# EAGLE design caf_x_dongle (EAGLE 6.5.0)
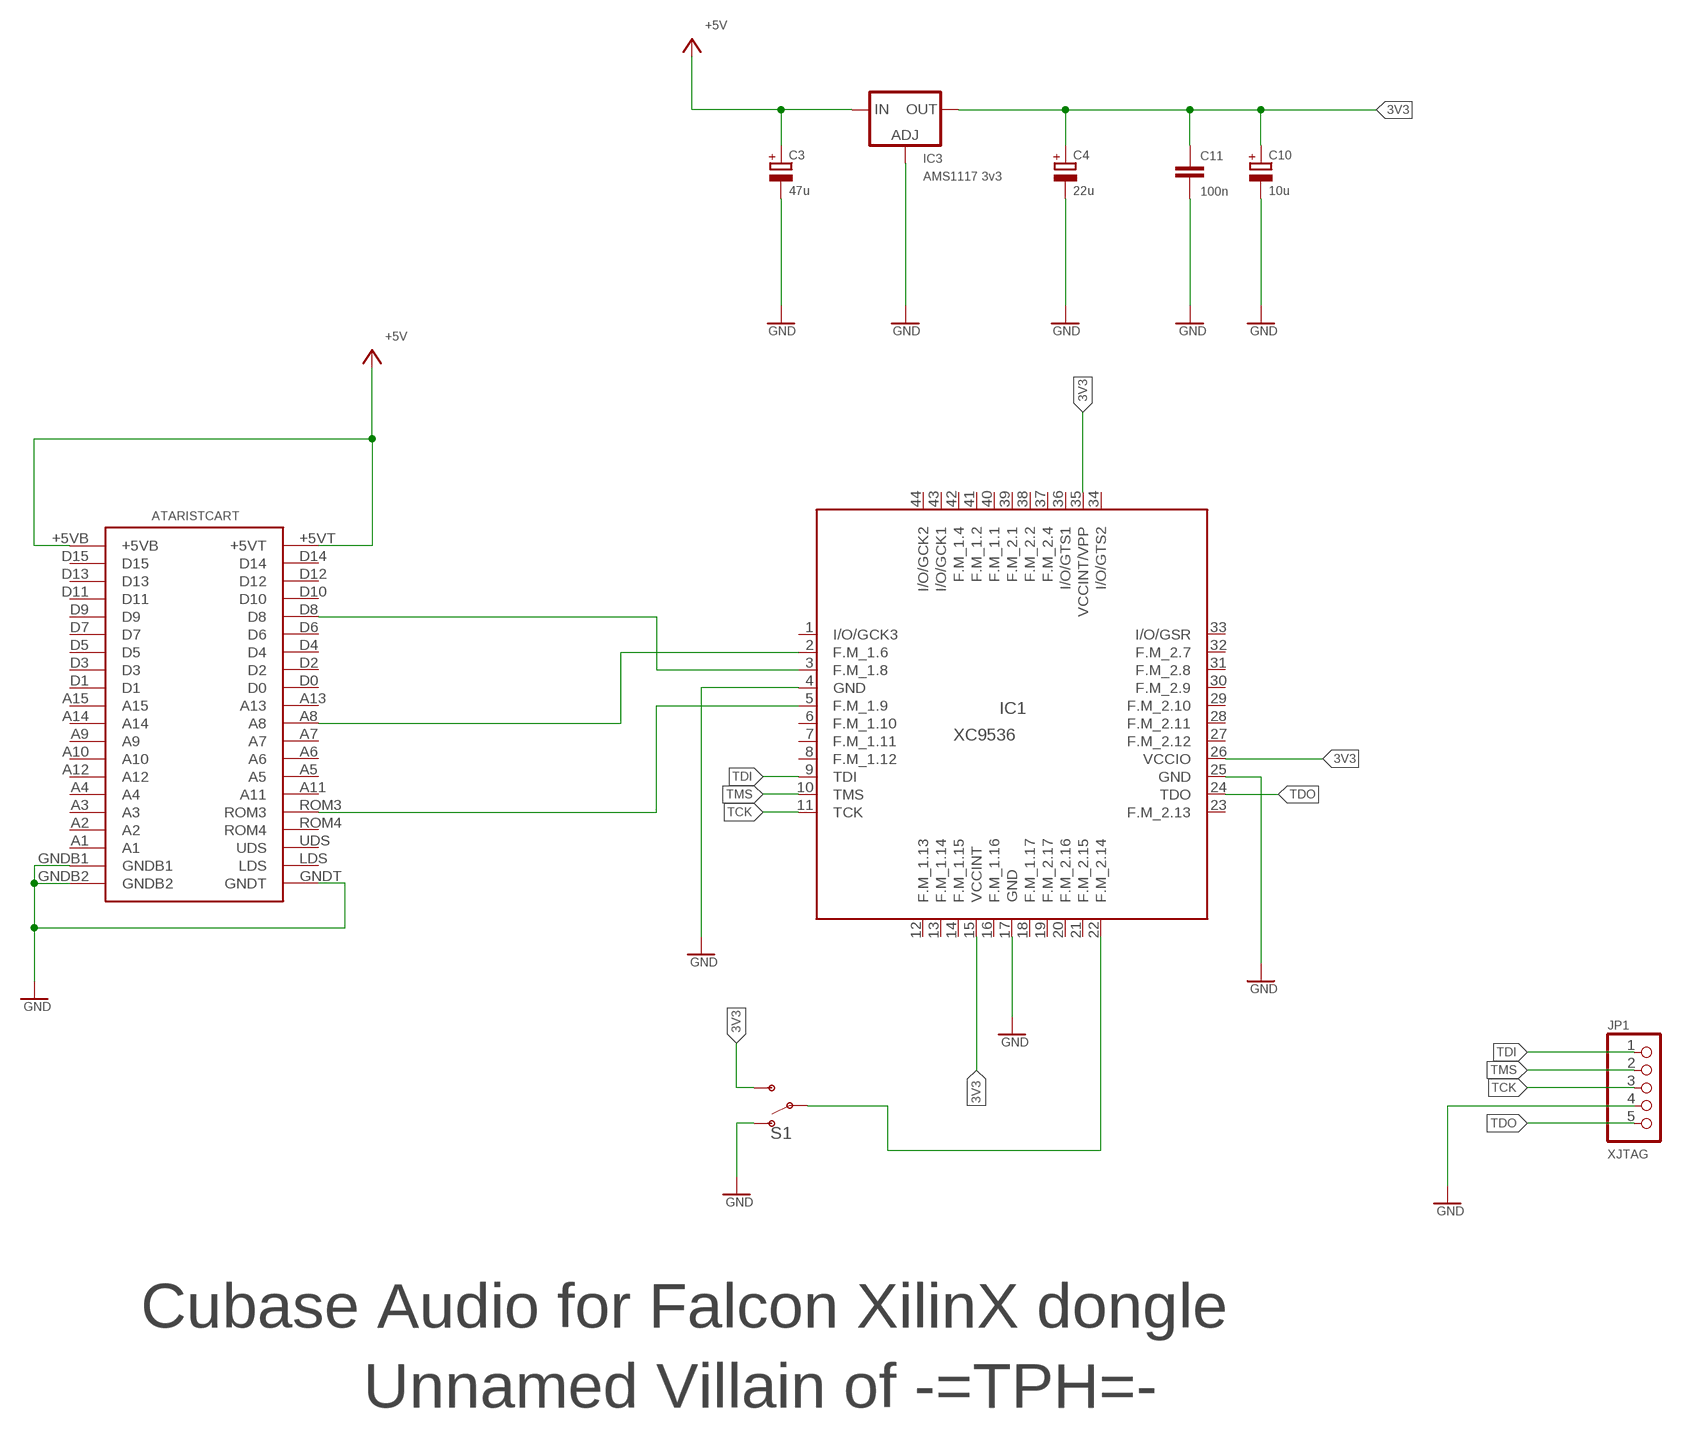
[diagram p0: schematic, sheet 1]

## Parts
C3  47u  CPOL-EUSMCD  [SMC_D]
C4  22u  CPOL-EUSMCD  [SMC_D]
C10  10u  CPOL-EUSMCB  [SMC_B]
C11  100n  C-EUC0805  [C0805]
IC1  XC9536  XC9536_44VQ  [SQFP-S-10X10-44]
IC3  AMS1117 3v3  LD117AS33TR  [SOT223]
JP1  XJTAG  PINHD-1X5  [1X05]
S1  SWITCH-SPDT-PTH-11.6X4.0MM-SHORT_LEADS  [SWITCH_SPDT_PTH_11.6X4.0MM]
U$1  ATARISTCART  [ATARISTCART]

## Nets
3V3: C4.+ C10.+ C11.1 IC1.15(VCCINT) IC1.26(VCCIO) IC1.35(VCCINT/VPP) IC3.4(OUT) S1.3(S)
+5V: C3.+ IC3.3(IN) U$1.+5VB U$1.+5VT
GND: C3.- C4.- C10.- C11.2 IC1.4(GND) IC1.17(GND) IC1.25(GND) IC3.1(ADJ) JP1.4 S1.1(O) U$1.GNDB1 U$1.GNDB2 U$1.GNDT
N$1: IC1.2(F.M_1.6) U$1.A8
N$2: IC1.3(F.M_1.8) U$1.D8
N$3: IC1.5(F.M_1.9) U$1.ROM3
N$4: IC1.22(F.M_2.14) S1.2(P)
TCK: IC1.11(TCK) JP1.3
TDI: IC1.9(TDI) JP1.1
TDO: IC1.24(TDO) JP1.5
TMS: IC1.10(TMS) JP1.2
Unconnected: IC1.1(I/O/GCK3) IC1.6(F.M_1.10) IC1.7(F.M_1.11) IC1.8(F.M_1.12) IC1.12(F.M_1.13) IC1.13(F.M_1.14) IC1.14(F.M_1.15) IC1.16(F.M_1.16) IC1.18(F.M_1.17) IC1.19(F.M_2.17) IC1.20(F.M_2.16) IC1.21(F.M_2.15) IC1.23(F.M_2.13) IC1.27(F.M_2.12) IC1.28(F.M_2.11) IC1.29(F.M_2.10) IC1.30(F.M_2.9) IC1.31(F.M_2.8) IC1.32(F.M_2.7) IC1.33(I/O/GSR) IC1.34(I/O/GTS2) IC1.36(I/O/GTS1) IC1.37(F.M_2.4) IC1.38(F.M_2.2) IC1.39(F.M_2.1) IC1.40(F.M_1.1) IC1.41(F.M_1.2) IC1.42(F.M_1.4) IC1.43(I/O/GCK1) IC1.44(I/O/GCK2) U$1.A1 U$1.A2 U$1.A3 U$1.A4 U$1.A5 U$1.A6 U$1.A7 U$1.A9 U$1.A10 U$1.A11 U$1.A12 U$1.A13 U$1.A14 U$1.A15 U$1.D0 U$1.D1 U$1.D2 U$1.D3 U$1.D4 U$1.D5 U$1.D6 U$1.D7 U$1.D9 U$1.D10 U$1.D11 U$1.D12 U$1.D13 U$1.D14 U$1.D15 U$1.LDS U$1.ROM4 U$1.UDS

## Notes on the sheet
- Cubase Audio for Falcon XilinX dongle
- Unnamed Villain of -=TPH=-

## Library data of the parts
C3 C4 C10 = rcl:CPOL-EU: POLARIZED CAPACITOR, European symbol
C11 = rcl:C-EU: CAPACITOR, European symbol
IC1 = xilinx-xc9500:XC9536_44VQ: xc9536_pc44 XC9500 In-System Programmable CPLD Family Auto generated by make-symbol-device-package-bsdl.ulp Rev. 34 Source: xc9536_vq44.bsd; MPN: XC9536-15VQG44C; OC_FARNELL: 1193227; OC_NEWARK: 98K3377
IC3 = v-reg:LD117A?*: Low drop fixed and adjustable positive voltage regulators 1 A Source: http://www.st.com/stonline/products/literature/ds/7194/ld1117axx.pdf
JP1 = pinhead:PINHD-1X5: PIN HEADER
S1 = SparkFun-Switches:SWITCH-SPDT: Single Pole, Double Throw (SPDT) Switch Single-pole, double-throw (SPDT) switch. Variant Overview SMD-AYZ0202 Surface Mount DPDT Switch (COM-00597) Used on e.g. LilyPad Arduino USB - ATmega32U4 Board PTH-11.6X4.0MM SPDT Mini Power Switch (COM-00102) Used on e.g. SparkFun Simon Says - Through-Hole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; PROD_ID: SWCH-13151
U$1 = Mq-AtariSTcart:ATARISTCART

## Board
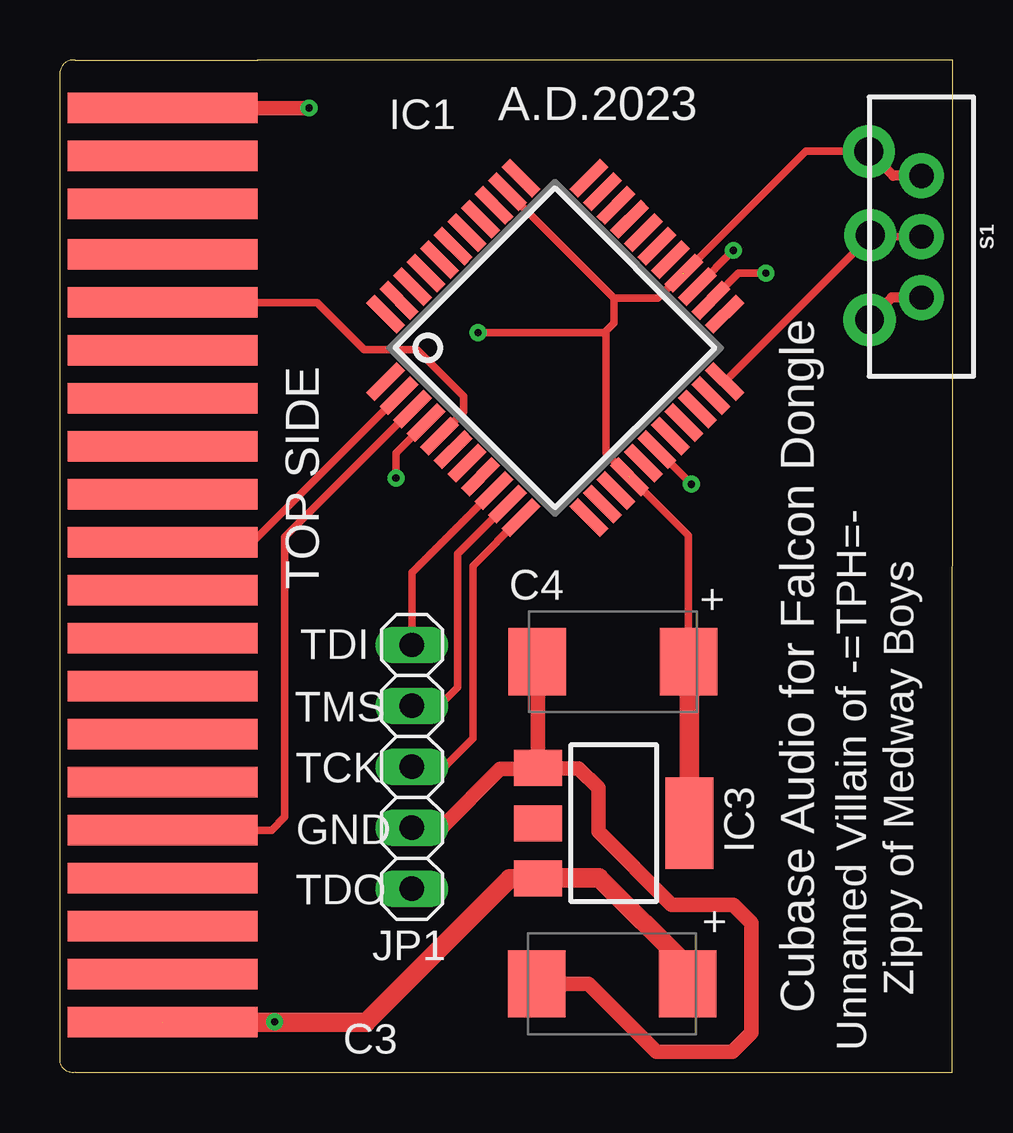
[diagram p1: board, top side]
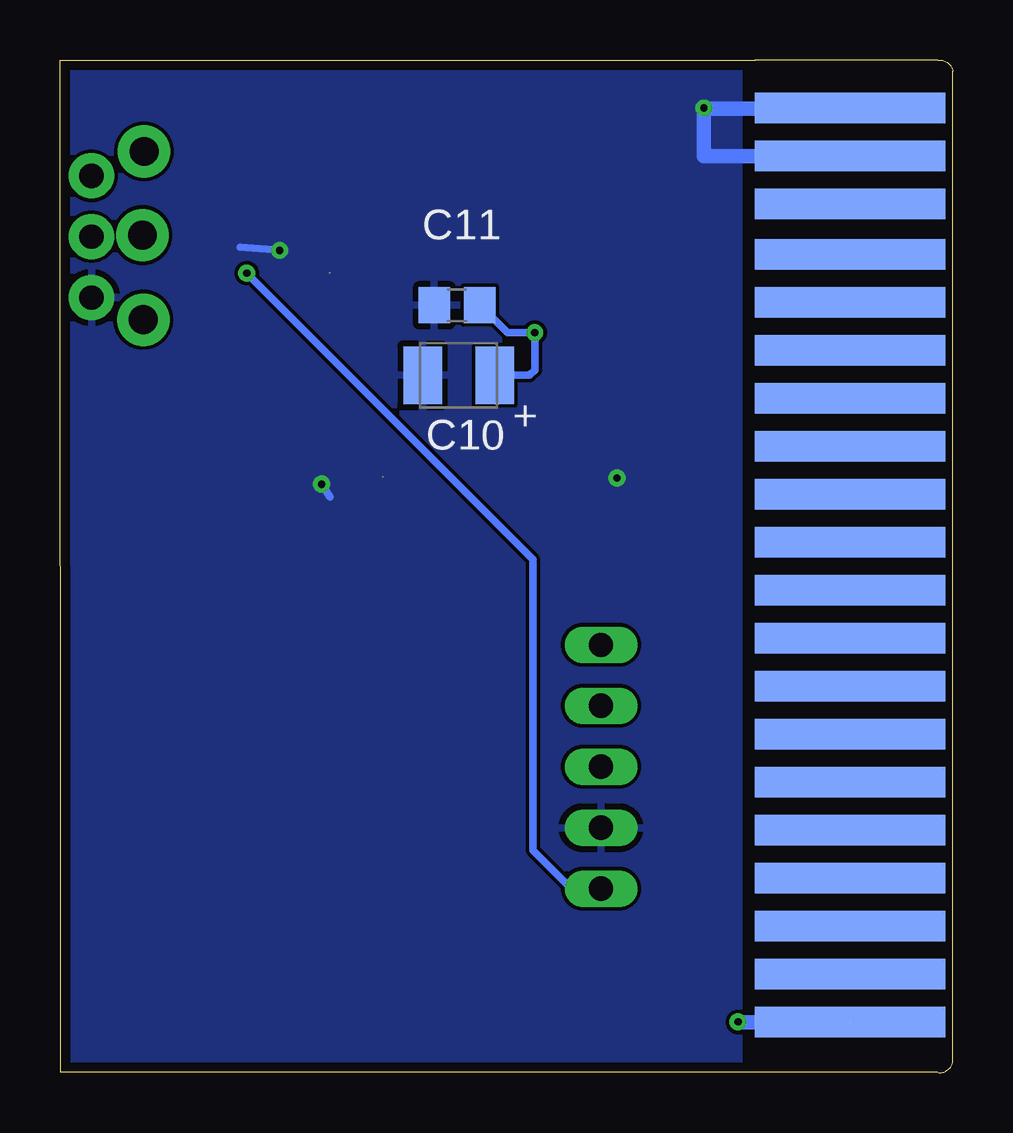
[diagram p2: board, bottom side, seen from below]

Size 37.22 x 42.21 mm. Coordinates in mm from the lower left corner, seen from the top.
Outline: 8.26,0.02 37.19,0.02 37.22,42.2 8.22,42.2
Copper layers (1*16): Top 0.035mm / dielectric 1.5mm / Bottom 0.035mm
Design rules "JLCPCB": minimum track width 5mil, minimum drill 8mil, track to track 6mil, track to pad 6mil, pad to pad 6mil, via to via 6mil, smd to smd 6mil, copper to edge 16mil, drill to drill 8mil, minimum pad ring 10mil, minimum via ring 8mil, stop-mask expansion 4mil, vias tented up to drill 0mil, thermal gap 10mil

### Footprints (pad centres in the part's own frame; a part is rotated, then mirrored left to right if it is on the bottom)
SMC_D = smd 2.4 x 2.8: + -3.15,0; - 3.15,0
SMC_B = smd 1.6 x 2.4: + -1.5,0; - 1.5,0
C0805 = smd 1.3 x 1.5: 1 -0.95,0; 2 0.95,0
SQFP-S-10X10-44 = smd 0.5 x 1.8: 1 -4,-6; 2 -3.2,-6; 3 -2.4,-6; 4 -1.6,-6; 5 -0.8,-6; 6 0,-6; 7 0.8,-6; 8 1.6,-6; 9 2.4,-6; 10 3.2,-6; 11 4,-6; 23 4,6; 24 3.2,6; 25 2.4,6; 26 1.6,6; 27 0.8,6; 28 0,6; 29 -0.8,6; 30 -1.6,6; 31 -2.4,6; 32 -3.2,6; 33 -4,6 | smd 1.8 x 0.5: 12 6,-4; 13 6,-3.2; 14 6,-2.4; 15 6,-1.6; 16 6,-0.8; 17 6,0; 18 6,0.8; 19 6,1.6; 20 6,2.4; 21 6,3.2; 22 6,4; 34 -6,4; 35 -6,3.2; 36 -6,2.4; 37 -6,1.6; 38 -6,0.8; 39 -6,0; 40 -6,-0.8; 41 -6,-1.6; 42 -6,-2.4; 43 -6,-3.2; 44 -6,-4
SOT223 = smd 1.5 x 2: 1 -2.3,-3.15; 2 0,-3.15; 3 2.3,-3.15 | smd 3.8 x 2: 4 0,3.15
1X05 = drill 1.016 long: 1 -5.08,0; 2 -2.54,0; 3 0,0; 4 2.54,0; 5 5.08,0
SWITCH_SPDT_PTH_11.6X4.0MM = drill 1.016 pad 1.88: 1 0,2.54; 2 0,0; 3 0,-2.54
ATARISTCART = smd 1.27 x 7.925 bottom: +5VB -19.31,-0.472; A1 14.79,-0.472; A2 12.69,-0.472; A3 10.69,-0.472; A4 8.69,-0.472; A9 2.69,-0.472; A10 4.69,-0.472; A12 6.69,-0.472; A14 0.69,-0.472; A15 -1.31,-0.472; D1 -3.31,-0.472; D3 -5.31,-0.472; D5 -7.31,-0.472; D7 -9.31,-0.472; D9 -11.31,-0.472; D11 -13.31,-0.472; D13 -15.31,-0.472; D15 -17.31,-0.472; GNDB1 16.79,-0.472; GNDB2 18.79,-0.472 | smd 1.27 x 7.925: +5VT -19.31,-0.472; A5 6.69,-0.472; A6 4.69,-0.472; A7 2.69,-0.472; A8 0.69,-0.472; A11 8.69,-0.472; A13 -1.31,-0.472; D0 -3.31,-0.472; D2 -5.31,-0.472; D4 -7.31,-0.472; D6 -9.31,-0.472; D8 -11.31,-0.472; D10 -13.31,-0.472; D12 -15.31,-0.472; D14 -17.31,-0.472; GNDT 18.79,-0.472; LDS 16.79,-0.472; ROM3 10.69,-0.472; ROM4 12.69,-0.472; UDS 14.79,-0.472

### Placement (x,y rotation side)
C3  23.02,3.7 180 top
C4  23.05,17.13 180 top
C10  20.61,29.07 180 bottom
C11  20.67,31.99 180 bottom
IC1  20.64,30.21 315 top
IC3  23.08,10.4 270 top
JP1  14.67,12.75 270 top
S1  35.91,34.85 180 top
U$1  3.81,21.42 90 top

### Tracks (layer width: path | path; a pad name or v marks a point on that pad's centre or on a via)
3V3  (via drill 0.3 pad 0.6)  (2 unrouted)
  Top 0.305: 33.72,38.4 31.09,38.4 IC1.26 | 25.97,33.32 24.92,32.28 23.1,32.28 | 23.1,32.28 23.1,31.25 22.7,30.85 | 22.7,30.85 v17.43,30.85 | C4.+ 26.2,22.39 IC1.15 22.77,25.83 22.77,30.78 22.7,30.85 | IC1.35 23.1,32.28
  Top 0.406: S1.3 34.73,37.39 33.72,38.4
  Top 0.813: IC3.4 26.23,17.1 C4.+
  Bottom 0.305: C11.1 18.58,30.85 v17.43,30.85 17.43,29.29 17.65,29.07 C10.+
+5V  (1 unrouted)
  Top 0.813: 26.2,3.67 C3.+ 26.17,4.42 22.48,8.11 19.95,8.11 IC3.3 19.91,8.08 18.73,8.08 12.76,2.11 U$1.+5VT
  Bottom 0.61: U$1.+5VT 8.95,2.11
GND  (via drill 0.3 pad 0.6)
  Top 0.305: v10.38,40.21 | IC1.4 14,25.83 v14,24.78 | IC1.25 v28.07,34.28 | IC1.17 v26.32,24.53
  Top 0.406: S1.1 34.67,32.31 33.72,31.36
  Top 0.61: JP1.4 15.91,10.21 18.35,12.65 19.89,12.65 IC3.1 | IC3.1 19.93,17.1 C4.- | U$1.GNDT v10.38,40.21 | C3.- 22.03,3.7 24.86,0.88 28.04,0.88 28.83,1.67 28.83,6.24 28.07,7 25.49,7 22.45,10.05 22.45,11.86 21.62,12.69 19.95,12.69 IC3.1
  Bottom 0.305: v10.38,40.21 10.35,40.21 | v28.07,34.28 29.72,34.4 | v26.32,24.53 25.97,23.99 | v14,24.78 13.97,24.78 v14,24.78
  Bottom 0.61: U$1.GNDB1 10.38,38.21 10.38,40.18 4.31,40.18 U$1.GNDT
  pour Bottom: 8.92,42.02 36.93,42.02 36.93,0.21 8.92,0.21
N$1
  Top 0.305: U$1.A8 8.01,22.11 IC1.2
N$2
  Top 0.305: U$1.D8 8.82,10.11 9.37,10.65 9.37,22.34 IC1.3
N$3
  Top 0.305: U$1.ROM3 10.71,32.11 12.67,30.15 14.89,30.15 16.83,28.21 16.83,27.53 IC1.5
N$4
  Top 0.305: S1.2 33.76,34.85 IC1.22
N$5  (via drill 1.2 pad 2.18)
  other vias: 33.78,34.91
N$6  (via drill 1.2 pad 2.18)
  other vias: 33.72,38.4
N$7  (via drill 1.2 pad 2.18)
  other vias: 33.75,31.39
N$8  (via drill 0.3 pad 0.6)
  other vias: 8.95,2.11
TCK
  Top 0.305: JP1.3 16.03,12.75 17.05,13.77 17.21,13.92 17.21,21.13 IC1.11
TDI
  Top 0.305: JP1.1 14.67,20.85 IC1.9
TDO  (via drill 0.3 pad 0.6)
  Top 0.305: v29.43,33.32 28.27,33.32 IC1.24
  Bottom 0.305: JP1.5 15.91,7.67 17.49,9.26 17.49,21.39 v29.43,33.32
TMS
  Top 0.305: JP1.2 15.81,15.29 16.57,16.05 16.57,21.62 IC1.10

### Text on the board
tNames: A.D.2023 | TOP SIDE | + | TDI | TMS | TCK | GND | TDO | + | Zippy of Medway Boys | Cubase Audio for Falcon Dongle | Unnamed Villain of -=TPH=-
bNames: +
